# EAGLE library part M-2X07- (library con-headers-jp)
MALE HEADER
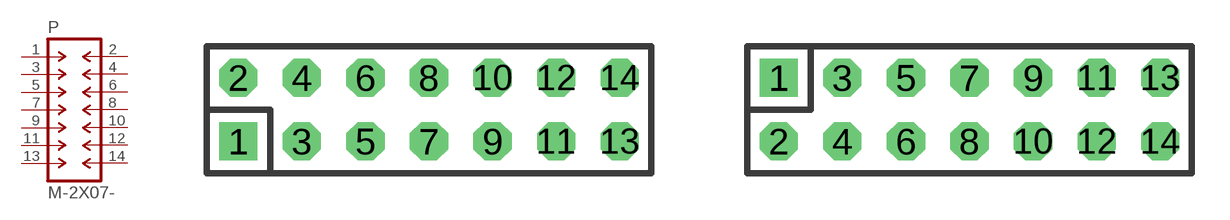
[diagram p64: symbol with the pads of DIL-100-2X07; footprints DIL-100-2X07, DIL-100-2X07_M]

Designator prefix P

## M-2X07-DIL-100  [DIL-100-2X07]
1  1  pas
2  2  pas
3  3  pas
4  4  pas
5  5  pas
6  6  pas
7  7  pas
8  8  pas
9  9  pas
10  10  pas
11  11  pas
12  12  pas
13  13  pas
14  14  pas

## M-2X07-DIL-100_M  [DIL-100-2X07_M]
Pads as for DIL-100-2X07

## M-2X07-DIL-2MM  [DIL-2MM-2X07]
Pads as for DIL-100-2X07

## M-2X07-DIL-2MM_M  [DIL-2MM-2X07_M]
Pads as for DIL-100-2X07

## M-2X07-87759  [87759-14]
Pads as for DIL-100-2X07

## M-2X07-87759_M  [87759-14_M]
Pads as for DIL-100-2X07

## Footprint DIL-100-2X07 (pad centres in mm)
PIN HEADER - 0.1"
drill 1.016 square: 1 -7.62,-1.27
drill 1.016 octagon: 2 -7.62,1.27; 3 -5.08,-1.27; 4 -5.08,1.27; 5 -2.54,-1.27; 6 -2.54,1.27; 7 0,-1.27; 8 0,1.27; 9 2.54,-1.27; 10 2.54,1.27; 11 5.08,-1.27; 12 5.08,1.27; 13 7.62,-1.27; 14 7.62,1.27

## Footprint DIL-100-2X07_M (pad centres in mm)
PIN HEADER - MIRRORED 0.1"
drill 1.016 square: 1 -7.62,1.27
drill 1.016 octagon: 2 -7.62,-1.27; 3 -5.08,1.27; 4 -5.08,-1.27; 5 -2.54,1.27; 6 -2.54,-1.27; 7 0,1.27; 8 0,-1.27; 9 2.54,1.27; 10 2.54,-1.27; 11 5.08,1.27; 12 5.08,-1.27; 13 7.62,1.27; 14 7.62,-1.27

## Footprint DIL-2MM-2X07 (pad centres in mm)
PIN HEADER - 2MM"
drill 0.711 square: 1 -6,-1
drill 0.711: 2 -6,1; 3 -4,-1; 4 -4,1; 5 -2,-1; 6 -2,1; 7 0,-1; 8 0,1; 9 2,-1; 10 2,1; 11 4,-1; 12 4,1; 13 6,-1; 14 6,1

## Footprint DIL-2MM-2X07_M (pad centres in mm)
PIN HEADER - MIRRORED 2MM
drill 0.711 square: 1 -6,1
drill 0.711: 2 -6,-1; 3 -4,1; 4 -4,-1; 5 -2,1; 6 -2,-1; 7 0,1; 8 0,-1; 9 2,1; 10 2,-1; 11 4,1; 12 4,-1; 13 6,1; 14 6,-1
